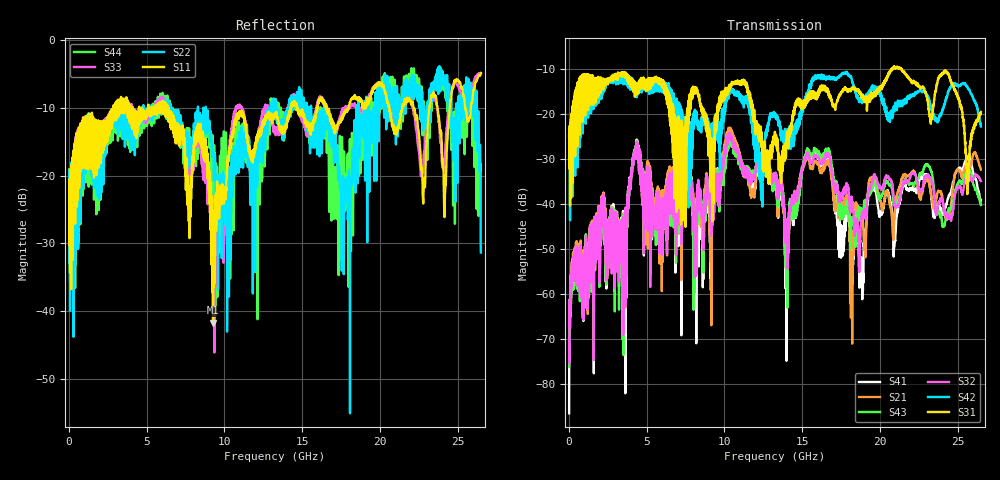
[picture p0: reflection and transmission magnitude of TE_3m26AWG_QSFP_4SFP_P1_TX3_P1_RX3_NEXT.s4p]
!Agilent Technologies,N5222A,MY51421691,A.10.00.00
!Agilent N5222A: A.10.00.00
!Date: Friday, January 30, 2015 12:34:36
!Correction: S11(Full 4 Port(1,2,3,4))
!S12(Full 4 Port(1,2,3,4))
!S13(Full 4 Port(1,2,3,4))
!S14(Full 4 Port(1,2,3,4))
!S21(Full 4 Port(1,2,3,4))
!S22(Full 4 Port(1,2,3,4))
!S23(Full 4 Port(1,2,3,4))
!S24(Full 4 Port(1,2,3,4))
!S31(Full 4 Port(1,2,3,4))
!S32(Full 4 Port(1,2,3,4))
!S33(Full 4 Port(1,2,3,4))
!S34(Full 4 Port(1,2,3,4))
!S41(Full 4 Port(1,2,3,4))
!S42(Full 4 Port(1,2,3,4))
!S43(Full 4 Port(1,2,3,4))
!S44(Full 4 Port(1,2,3,4))
!S4P File: Measurements: <S11,S12,S13,S14>,
!<S21,S22,S23,S24>,
!<S31,S32,S33,S34>,
!<S41,S42,S43,S44>:
# Hz S  dB  R 50.0
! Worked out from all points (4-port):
!   2650 points, 10 MHz to 26.5 GHz, reference 50 ohm
!   strongest paths, dB at 10 MHz, 6.63 GHz, 13.26 GHz, 19.88 GHz, 26.5 GHz:
!     S31: -24.9, -17.8, -24.7, -15.3, -19.6
!     S42: -25.0, -15.8, -19.9, -14.1, -22.8
!     S32: -70.7, -38.3, -33.7, -35.7, -34.9
!     S43: -76.2, -38.9, -34.6, -38.1, -40.3
!     S21: -61.5, -36.5, -34.7, -37.4, -32.4
!     S41: -86.6, -37.2, -34.8, -40.5, -39.3
!   lowest |S11| = -41.8 dB at 9.27 GHz (marker M1), VSWR 1.02, Z = 50.1 + j0.81 ohm
!   |S11| at or under -10 dB: start of sweep to 2.858 GHz; 6.4 GHz to 14.25 GHz (7.85 GHz wide, 76 % of centre); 16.59 GHz to 17.99 GHz (1.399 GHz wide, 8.09 % of centre)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
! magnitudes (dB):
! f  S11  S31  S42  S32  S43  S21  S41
! 10 MHz  -20.8  -24.9  -25.0  -70.7  -76.2  -61.5  -86.6
! 4.33 GHz  -10.6  -14.0  -14.6  -28.2  -28.1  -27.9  -27.8
! 9.27 GHz  -41.8  -27.7  -22.0  -42.7  -41.6  -39.8  -39.7
! 10.86 GHz  -11.2  -13.0  -15.6  -28.0  -28.5  -27.6  -28.1
! 18.2 GHz  -8.6  -14.3  -12.4  -38.6  -43.9  -51.7  -62.4
! 23.93 GHz  -13.7  -11.5  -20.4  -38.8  -42.6  -37.2  -40.9
! 26.5 GHz  -4.8  -19.6  -22.8  -34.9  -40.3  -32.4  -39.3
